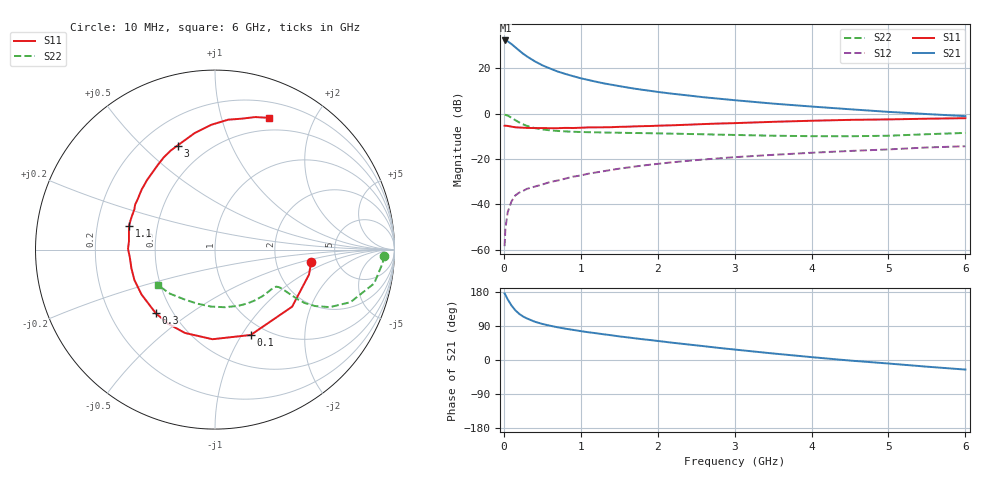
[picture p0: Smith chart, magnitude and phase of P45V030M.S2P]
! SIEMENS Small Signal Semiconductors
! BFP182
! Si NPN RF Bipolar Junction Transistor in SOT143
! VCE = 5 V  IC = 30 mA
! Common Emitter S-Parameters:  March  1996
# GHz  S  MA  R  50
!  f  S11  S21  S12  S22
! GHz  MAG  ANG  MAG  ANG  MAG  ANG  MAG  ANG
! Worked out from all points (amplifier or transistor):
!   36 points, 10 MHz to 6 GHz, reference 50 ohm
!   highest |S21| = 32.2 dB at 20 MHz (marker M1)
!   |S21| within 3 dB of that: start of sweep to 149.2 MHz
!   unconditionally stable (mu >= 1): 612.6 MHz to 5.488 GHz
!   at 250 MHz: K = 0.60, MSG = 30.2 dB, |S12| = -34.1 dB
!   at 1.4 GHz: K = 1.22, MAG = 15.9 dB, |S12| = -24.8 dB
!   at 6 GHz: K = 0.95, MSG = 6.6 dB, |S12| = -14.4 dB
!   S11 on the Smith chart (normalised r, x): 10 MHz: 3.22, -0.62; 100 MHz: 0.85, -1.10; 300 MHz: 0.40, -0.37; 1.1 GHz: 0.34, +0.12; 3 GHz: 0.35, +0.65; 6 GHz: 0.36, +1.42
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0.01  0.5403 -7.2  40.87 175.6  0.0012 84.0  0.9435 -2.0
0.02  0.5419 -14.9  40.88 172.0  0.0029 87.1  0.9366 -4.7
0.05  0.5346 -36.5  39.24 160.1  0.0067 74.5  0.9066 -12.0
0.1  0.5156 -67.3  33.98 143.7  0.0117 64.1  0.8098 -21.2
0.15  0.4995 -91.6  28.87 131.0  0.0158 57.7  0.7161 -26.6
0.2  0.4937 -109.8  24.5 121.7  0.0182 55.2  0.6384 -29.5
0.25  0.4885 -122.4  20.89 114.9  0.0198 52.9  0.5798 -30.8
0.3  0.4843 -133.0  18.2 109.7  0.022 52.5  0.5371 -31.0
0.4  0.4797 -148.5  14.27 101.2  0.0246 53.3  0.4803 -30.7
0.5  0.48 -159.3  11.6 95.2  0.0274 52.7  0.4478 -30.4
0.6  0.4772 -167.4  9.865 90.5  0.031 54.4  0.4281 -30.3
0.7  0.4766 -174.8  8.447 86.3  0.0336 55.9  0.4146 -30.4
0.9  0.4815 174.5  6.682 79.5  0.0408 56.6  0.3981 -31.3
1.1  0.4965 164.9  5.499 73.2  0.0475 56.8  0.3894 -33.3
1.3  0.4993 157.8  4.637 67.8  0.0539 56.6  0.3829 -35.7
1.6  0.5143 146.7  3.779 59.9  0.0645 55.4  0.3757 -40.1
2.2  0.5532 129.1  2.729 45.4  0.0849 51.4  0.3619 -50.7
3  0.6163 109.8  1.974 27.6  0.1097 44.5  0.3388 -68.0
3.5  0.6591 99.9  1.661 17.2  0.1234 39.9  0.3255 -80.5
4.5  0.7276 84.2  1.246 -1.5  0.1503 31.2  0.317 -108.3
5.5  0.7717 73.1  0.977 -17.6  0.1793 22.9  0.3513 -135.7
6  0.7926 67.9  0.879 -25.3  0.191 17.8  0.3756 -148.5
